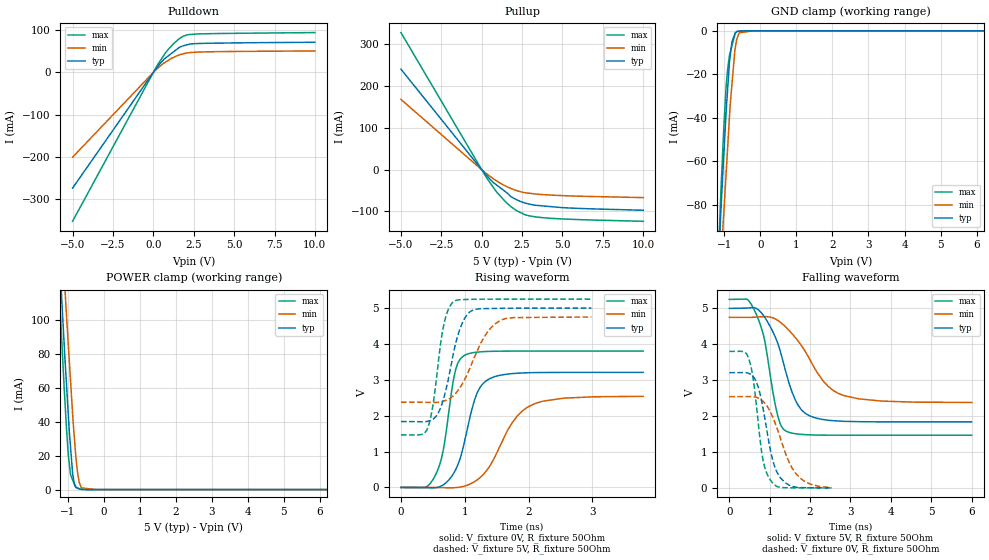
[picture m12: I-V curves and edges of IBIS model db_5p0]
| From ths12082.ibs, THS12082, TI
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|   db_5p0 Model
[Model]   db_5p0
Model_type   I/O
Polarity   Non-Inverting
Enable   Active-High
Vinl = 0.6
Vinh = 2.6
Vmeas = 2.5
Vref = 2.5
Cref = 30pF
Rref = 50
|   typ   min   max
|   (nom PVT)   (fast PVT)   (slow PVT)
C_comp   1.747e-12   1.738e-12   1.778e-12
|ON state : BUFFER OUTPUT TURNED HIGH
|C_comp   1.893e-12   1.883e-12   1.946e-12
|OFF state: BUFFER IN HIGH IMPEDANCE
|C_comp   1.601e-12   1.593e-12   1.609e-12
| Where nom  PVT is Nominal Process, 5V, 27C
|   Fast PVT is Strong Process,  5.25V, -55C
|   Slow PVT is Weak Process,   4.75V, 125C
[Voltage Range]   5   4.75   5.25
|Ambient Temperature   25   125   -55
|Junction Temperature
[Temperature Range]   27   125   -55
[Pullup Reference]   5   4.75   5.25
[Pulldown Reference]   0   0   0
[Power Clamp Reference]   5   4.75   5.25
[GND Clamp Reference]   0   0   0
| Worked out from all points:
|   slope of the pulldown table from 0 to 0.75 V, typ, clamps not added: 21.9 ohm
|   slope of the pullup table from 0 to 0.75 V, typ, clamps not added: 23.7 ohm
|   GND clamp passes 1 mA (typ) near -0.70 V on its own axis
|   POWER clamp passes 1 mA (typ) near -0.76 V on its own axis
|   falling waveform, V_fixture 5V, R_fixture 50Ohm: 20-80 % time 555ps typ, 859ps min, 372ps max; typ from 5 V to 1.84 V
|   rising waveform, V_fixture 0V, R_fixture 50Ohm: 20-80 % time 286ps typ, 488ps min, 200ps max; typ from 0 V to 3.21 V
|   rising waveform, V_fixture 5V, R_fixture 50Ohm: 20-80 % time 246ps typ, 385ps min, 172ps max; typ from 1.84 V to 5 V
|   falling waveform, V_fixture 0V, R_fixture 50Ohm: 20-80 % time 336ps typ, 527ps min, 248ps max; typ from 3.21 V to 0.001 V
[Pulldown]
|   Voltage   I(typ)   I(min)   I(max)
-5V       -273.8mA   -200.7mA   -352.4mA
283.5mV   14.69mA    10.52mA    19.52mA
700mV     32.81mA    23.07mA    43.39mA
924mV     39.34mA    28.46mA    54.61mA
1.286V    49.89mA    36.37mA    69.5mA
1.596V    58.91mA    41.32mA    79.62mA
1.827V    62.89mA    43.91mA    85.41mA
2.111V    65.66mA    46.32mA    89.26mA
2.594V    68.16mA    47.96mA    90.97mA
10V       71.52mA    50.93mA    94.44mA
[GND Clamp]
|   Voltage   I(typ)   I(min)   I(max)
-5V       -1.744A    -1.639A    -1.893A
-1.306V   -157.1mA   -175.8mA   -159.5mA
-1.092V   -81.23mA   -106.4mA   -72.03mA
-1.04V    -64.65mA   -90.47mA   -53.21mA
-950.3mV  -36.78mA   -65.1mA    -25.38mA
-855mV    -13.69mA   -38.26mA   -10.86mA
-790mV    -5.114mA   -24.59mA   -6.842mA
-712.5mV  -1.548mA   -9.457mA   -2.047mA
-640.5mV  -260uA     -3.089mA   -190.7uA
-589mV    -196.5uA   -904.1uA   -175.4uA
-190mV    0A         -26.17nA   -56.58uA
10V       0A         0A         0A
[Pullup]
|   Voltage   I(typ)   I(min)   I(max)
-5V       240.8mA    168.3mA    328.5mA
294mV     -13.42mA   -9.454mA   -18.95mA
700mV     -30.18mA   -21.2mA    -41.41mA
924mV     -36.77mA   -26.8mA    -53.46mA
1.507V    -53.92mA   -39.84mA   -78.24mA
1.822V    -64.83mA   -45.16mA   -88.88mA
2.163V    -72.02mA   -50.18mA   -98.28mA
2.678V    -79.75mA   -55.13mA   -107.9mA
3.36V     -85.35mA   -58.46mA   -113.3mA
5.405V    -91.76mA   -62.72mA   -118.6mA
10V       -97.14mA   -66.87mA   -123.7mA
[POWER Clamp]
|   Voltage   I(typ)   I(min)   I(max)
-5V       1.846A     1.827A     1.872A
-1.306V   168.4mA    207.4mA    147.2mA
-1.103V   87.71mA    128.7mA    62.29mA
-1.08V    78.9mA     120.2mA    53.79mA
-1.034V   62.66mA    103.3mA    36.71mA
-981.8mV  44.03mA    85.25mA    20.18mA
-918.7mV  24.76mA    63.74mA    8.72mA
-860mV    9.326mA    43.68mA    5.584mA
-815mV    3.518mA    30.69mA    3.182mA
-731.5mV  811.4uA    11.12mA    1.116mA
-640mV    112.2uA    2.178mA    202uA
10V       0A         0A         0A
[Ramp]
R_load = 50
|   typ   min   max
dV/dt_r   1.92509/2.84791e-10   1.52411/4.85172e-10   2.28107/1.99197e-10
dV/dt_f   1.89778/5.54678e-10   1.42247/8.56677e-10   2.27014/3.70788e-10
[Falling Waveform]
V_fixture = 5V
V_fixture_min = 4.75V
V_fixture_max = 5.25V
R_fixture = 50Ohm
|   Time   V(typ)   V(min)   V(max)
0s        5V         4.75V      5.25V
436ps     5.007V     4.749V     5.258V
674ps     4.994V     4.757V     4.82V
874ps     4.756V     4.769V     4.114V
1.192ns   4.05V      4.67V      2.041V
1.4ns     3.227V     4.477V     1.583V
1.87ns    2.085V     3.821V     1.483V
2.35ns    1.899V     2.944V     1.469V
2.796ns   1.856V     2.587V     1.467V
6ns       1.837V     2.379V     1.466V
[Rising Waveform]
V_fixture = 0V
V_fixture_min = 0V
V_fixture_max = 0V
R_fixture = 50Ohm
|   Time   V(typ)   V(min)   V(max)
0s        1.848nV    2.664nV    1.571nV
546ps     -6.901mV   -2.511mV   361.1mV
664ps     72.62mV    -6.27mV    1.048V
852ps     476.6mV    -5.889mV   3.245V
984ps     1.179V     31.19mV    3.669V
1.198ns   2.649V     215.4mV    3.773V
1.398ns   3.038V     608.4mV    3.794V
1.75ns    3.175V     1.82V      3.801V
2.102ns   3.201V     2.338V     3.801V
3.798ns   3.208V     2.54V      3.802V
[Rising Waveform]
V_fixture = 5V
V_fixture_min = 4.75V
V_fixture_max = 5.25V
R_fixture = 50Ohm
|   Time   V(typ)   V(min)   V(max)
0s        1.837V     2.378V     1.466V
418ps     1.844V     2.371V     1.652V
502ps     1.903V     2.367V     2.296V
672ps     2.493V     2.408V     4.536V
822ps     3.736V     2.559V     5.18V
922ps     4.408V     2.772V     5.231V
1.06ns    4.863V     3.24V      5.242V
1.334ns   4.986V     4.274V     5.248V
1.558ns   4.994V     4.656V     5.249V
2.986ns   5V         4.75V      5.25V
[Falling Waveform]
V_fixture = 0V
V_fixture_min = 0V
V_fixture_max = 0V
R_fixture = 50Ohm
|   Time   V(typ)   V(min)   V(max)
0s        3.209V     2.54V      3.802V
370ps     3.211V     2.542V     3.787V
488ps     3.186V     2.544V     3.578V
602ps     3.085V     2.539V     2.953V
736ps     2.732V     2.492V     1.6V
844ps     2.164V     2.4V       721.1mV
1.06ns    836mV      2.011V     151.4mV
1.274ns   268.3mV    1.353V     10.18mV
1.646ns   18.07mV    399.7mV    1.585mV
2.528ns   803.5uV    6.362mV    215.2uV
